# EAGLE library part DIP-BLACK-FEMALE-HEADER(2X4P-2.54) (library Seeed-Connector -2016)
320030087
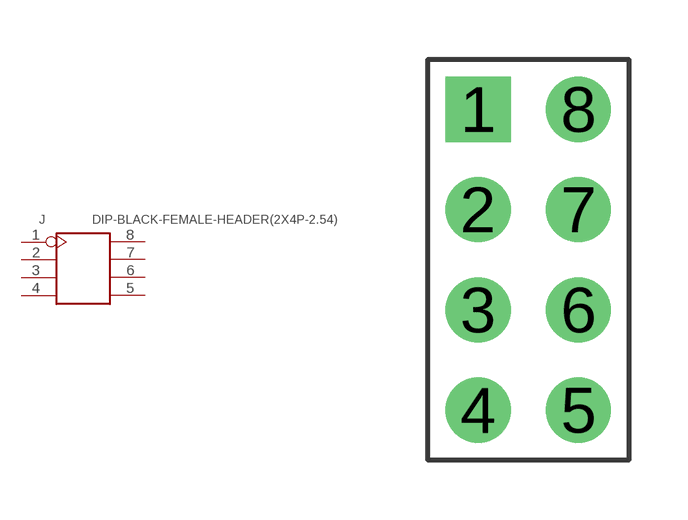
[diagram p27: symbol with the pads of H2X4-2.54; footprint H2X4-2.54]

Designator prefix J

## DIP-BLACK-FEMALE-HEADER(2X4P-2.54) (VALUE: 2X4P-2.54)  [H2X4-2.54]
1  1
2  2
3  3
4  4
5  5
6  6
7  7
8  8

## Footprint H2X4-2.54 (pad centres in mm)
drill 0.889 pad 1.651 square: 1 -1.27,3.81
drill 0.889 pad 1.651: 2 -1.27,1.27; 3 -1.27,-1.27; 4 -1.27,-3.81; 5 1.27,-3.81; 6 1.27,-1.27; 7 1.27,1.27; 8 1.27,3.81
